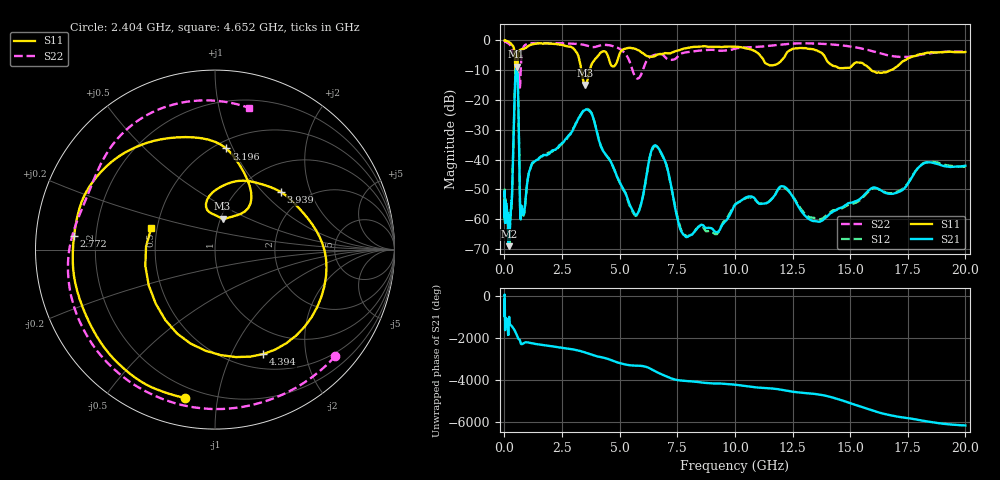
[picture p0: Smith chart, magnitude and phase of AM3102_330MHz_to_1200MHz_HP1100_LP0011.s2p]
! Date/Time: Tue, Sep 11, 2018 5:21 PM
! Network Analyzer: Agilent Technologies E8362B Rev: A.07.50.63
! Sweep from 0.010 to 20.000 GHz, 1601 Points, Sweep Type: LOG
! Power Supply: 4.949 V, 0.001 A
# Hz S DB R 50
!freq MagS11 AngS11 MagS21 AngS21 MagS12 AngS12 MagS22 AngS22
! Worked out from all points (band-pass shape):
!   1601 points, 10 MHz to 20 GHz, reference 50 ohm
!   highest |S21| = -8.87 dB at 528.1 MHz (marker M1); lowest = -69.1 dB at 185.7 MHz (marker M2)
!   |S21| within 3 dB of the highest: 476.8 MHz to 571.7 MHz (94.84 MHz wide, 18.1 % of centre)
!   lowest |S11| = -15.0 dB at 3.498 GHz (marker M3), VSWR 1.43, Z = 51.1 + j18.3 ohm
!   |S11| at or under -10 dB: 472.4 MHz to 527.4 MHz (54.94 MHz wide, 11 % of centre); 3.34 GHz to 3.701 GHz (361 MHz wide, 10.3 % of centre); 15.91 GHz to 16.77 GHz (851.9 MHz wide, 5.21 % of centre)
!   |S22| runs from -15.8 to -0.2 dB; largest |S21 - S12| = 0.0047
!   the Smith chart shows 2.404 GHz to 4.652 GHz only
!   S11 on the Smith chart (normalised r, x): 2.404 GHz: 0.14, -0.81; 2.772 GHz: 0.12, +0.05; 3.196 GHz: 0.57, +0.94; 3.939 GHz: 1.51, +1.27; 4.394 GHz: 0.68, -1.33; 4.652 GHz: 0.46, +0.13
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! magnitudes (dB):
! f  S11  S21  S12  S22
! 10 MHz  0.0  -52.3  -50.1  -0.2
! 35.55 MHz  -0.1  -59.5  -57.8  -0.3
! 126.4 MHz  -0.3  -58.4  -58.7  -0.8
! 185.7 MHz  -0.5  -69.1  -65.2  -1.1
! 322.2 MHz  -1.5  -53.8  -53.7  -3.1
! 447.2 MHz  -4.5  -18.2  -18.2  -4.3
! 528.1 MHz  -10.0  -8.9  -8.9  -9.2
! 591.9 MHz  -5.9  -16.7  -16.8  -11.4
! 702.3 MHz  -3.1  -59.9  -59.2  -11.7
! 1.59 GHz  -1.0  -39.0  -39.0  -0.9
! 2.404 GHz  -1.5  -35.1  -35.5  -1.0
! 2.772 GHz  -2.1  -32.1  -32.4  -1.0
! 3.196 GHz  -4.9  -26.3  -26.5  -1.2
! 3.498 GHz  -15.0  -23.4  -23.3  -1.6
! 3.939 GHz  -6.2  -28.4  -28.4  -2.2
! 4.394 GHz  -3.9  -38.3  -38.3  -1.5
! 4.652 GHz  -8.5  -41.3  -41.3  -1.8
! 5.652 GHz  -2.8  -58.3  -58.6  -11.9
! 6.58 GHz  -5.0  -35.3  -35.5  -4.7
! 7.958 GHz  -2.5  -65.9  -65.8  -3.9
! 13.68 GHz  -3.9  -60.9  -60.1  -1.1
! 20 GHz  -3.9  -42.1  -42.5  -3.7
